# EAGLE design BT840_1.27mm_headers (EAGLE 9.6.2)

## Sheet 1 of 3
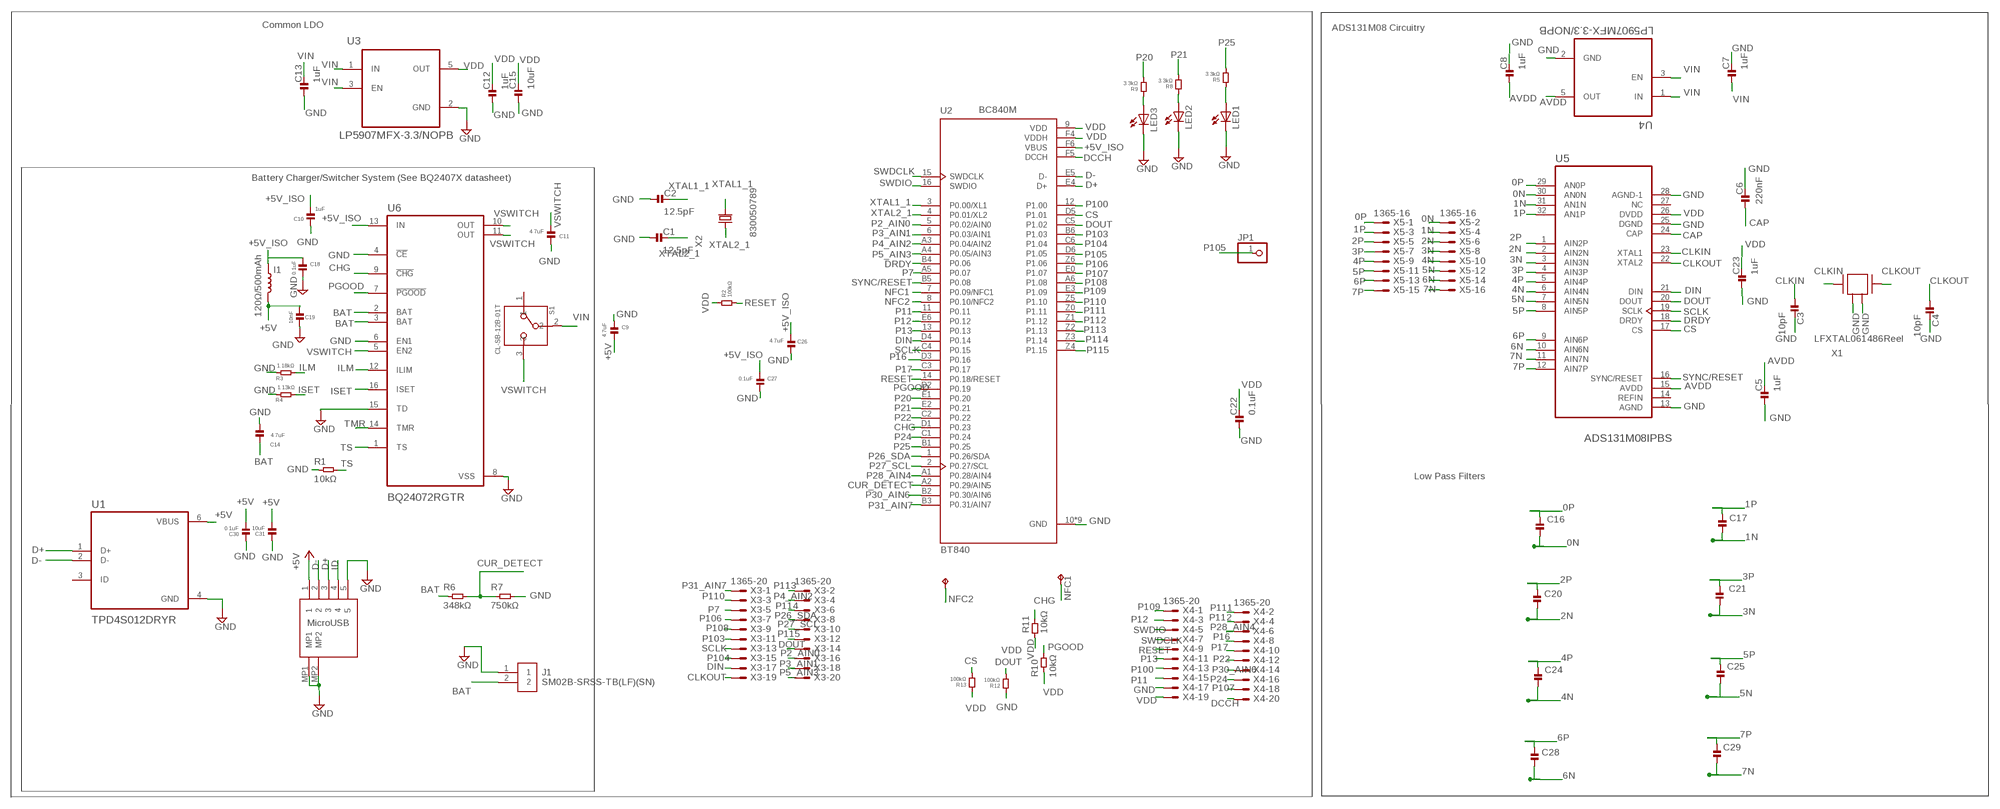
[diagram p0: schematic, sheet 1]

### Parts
C1  12.5pF  CAPACITOR.0201  [0201]
C2  12.5pF  CAPACITOR.0201  [0201]
C3  10pF  CAPACITOR.0201  [0201]
C4  10pF  CAPACITOR.0201  [0201]
C5  1uF  CAPACITOR.0201  [0201]
C6  220nF  CAPACITOR.0201  [0201]
C7  1uF  CAPACITOR.0201  [0201]
C8  1uF  CAPACITOR.0201  [0201]
C9  4.7uF  CAPACITOR.0201  [0201]
C10  1uF  CAPACITOR.0201  [0201]
C11  4.7uF  CAPACITOR.0201  [0201]
C12  1uF  CAPACITOR.0201  [0201]
C13  1uF  CAPACITOR.0201  [0201]
C14  4.7uF  CAPACITOR.0201  [0201]
C15  10uF  CAPACITOR.0402  [0402]
C16  100pF  CAPACITOR.0201  [0201]
C17  100pF  CAPACITOR.0201  [0201]
C18  0.1uF  CAPACITOR.0201  [0201]
C19  10nF  CAPACITOR.0201  [0201]
C20  100pF  CAPACITOR.0201  [0201]
C21  100pF  CAPACITOR.0201  [0201]
C22  0.1uF  CAPACITOR.0201  [0201]
C23  1uF  CAPACITOR.0201  [0201]
C24  100pF  CAPACITOR.0201  [0201]
C25  100pF  CAPACITOR.0201  [0201]
C26  4.7uF  CAPACITOR.0201  [0201]
C27  0.1uF  CAPACITOR.0201  [0201]
C28  100pF  CAPACITOR.0201  [0201]
C29  100pF  CAPACITOR.0201  [0201]
C30  0.1uF  CAPACITOR.0201  [0201]
C31  10uF  CAPACITOR.0402  [0402]
I1  120Ω/500mAh  12NH-0402  [0402_COILCRAFT]
J1  SM02B-SRSS-TB(LF)(SN)  [SM02B-SRSS-TB(LF)(SN)]
JP1  PINHD-1X1  [1X01]
LED1  LEDCHIPLED_0603  [CHIPLED_0603]
LED2  LEDCHIPLED_0603  [CHIPLED_0603]
LED3  LEDCHIPLED_0603  [CHIPLED_0603]
NFC1  TPTP14SQ  [TP14SQ]
NFC2  TPTP14SQ  [TP14SQ]
R1  10kΩ  RESISTOR.0201  [0201]
R2  100kΩ  RESISTOR.0201  [0201]
R3  1.18kΩ  RESISTOR.0201  [0201]
R4  1.13kΩ  RESISTOR.0201  [0201]
R5  3.3kΩ  RESISTOR.0201  [0201]
R6  348kΩ  RESISTOR.0201  [0201]
R7  750kΩ  RESISTOR.0201  [0201]
R8  3.3kΩ  RESISTOR.0201  [0201]
R9  3.3kΩ  RESISTOR.0201  [0201]
R10  10kΩ  RESISTOR.0402  [0402]
R11  10kΩ  RESISTOR.0402  [0402]
R12  100kΩ  RESISTOR.0402  [0402]
R13  100kΩ  RESISTOR.0402  [0402]
S1  CL-SB-12B-01T  [CL-SB-12B]
U1  TPD4S012DRYR  [PSON50P145X100X60-6N]
U2  BT840  [XCVR_BT840]
U3  LP5907MFX-3.3/NOPB  [SOT95P280X145-5N]
U4  LP5907MFX-3.3/NOPB  [SOT95P280X145-5N]
U5  ADS131M08IPBS  [QFP50P700X700X120-32N]
U6  BQ24072RGTR  [QFN50P300X300X100-17N]
U7  DX4R005JJ2R1800  [DX4R005JJ2R1800]
X1  ABM3B-8.000MHZ-B2-T  [ABM3B-8.000MHZ-B2-T]
X2  FC-12M  [FC-12M]
X3  1365-20  [1365-20]
X4  1365-20  [1365-20]
X5  1365-16  [1365-16]

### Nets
0N: C16.2 U5.30(AN0N) X5.2
0P: C16.1 U5.29(AN0P) X5.1
1N: C17.2 U5.31(AN1N) X5.4
1P: C17.1 U5.32(AN1P) X5.3
2N: C20.2 U5.2(AIN2N) X5.6
2P: C20.1 U5.1(AIN2P) X5.5
3N: C21.2 U5.3(AIN3N) X5.8
3P: C21.1 U5.4(AIN3P) X5.7
4N: C24.2 U5.6(AIN4N) X5.10
4P: C24.1 U5.5(AIN4P) X5.9
5N: C25.2 U5.7(AIN5N) X5.12
5P: C25.1 U5.8(AIN5P) X5.11
6N: C28.2 U5.10(AIN6N) X5.14
6P: C28.1 U5.9(AIN6P) X5.13
7N: C29.2 U5.11(AIN7N) X5.16
7P: C29.1 U5.12(AIN7P) X5.15
+5V: C9.2 C19.2 C30.2 C31.2 I1.P$2 U1.6(VBUS) U7.1
+5V_ISO: C10.2 C18.1 C26.2 C27.2 I1.P$1 U2.F6(VBUS) U6.13(IN)
AVDD: C5.2 C8.1 U4.5(OUT) U5.15(AVDD)
BAT: C14.2 J1.2 R6.1 U6.2(BAT) U6.3(BAT)
CAP: C6.1 U5.24(CAP)
CHG: R11.2 U2.D1(P0.23) U6.9(!CHG)
CLKIN: C3.1 U5.23(XTAL1) X1.1
CLKOUT: C4.1 U5.22(XTAL2) X1.3 X3.19
CS: R13.1 U2.D5(P1.01) U5.17(CS)
CUR_DETECT: R6.2 R7.1 U2.A2(P0.29/AIN5)
D+: U1.1(D+) U2.E4(D+) U7.3
D-: U1.2(D-) U2.E5(D-) U7.2
DCCH: U2.F5(DCCH) X4.20
DIN: U2.D4(P0.14) U5.21(DIN) X3.17
DOUT: R12.1 U2.C5(P1.02) U5.20(DOUT) X3.14
DRDY: U2.B4(P0.06) U5.18(DRDY)
GND: C1.1 C2.1 C3.2 C4.2 C5.1 C6.2 C7.2 C8.2 C9.1 C10.1 C11.1 C12.1 C13.1 C14.1 C15.1 C18.2 C19.1 C22.1 C23.1 C26.1 C27.1 C30.1 C31.1 J1.1 LED1.C LED2.C LED3.C R1.1 R3.1 R4.1 R7.2 R12.2 U1.4(GND) U2.10(GND) U2.A0(GND) U2.B0(GND) U2.C0(GND) U2.D0(GND) U2.F0(GND) U2.F1(GND) U2.F2(GND) U2.F3(GND) U3.2(GND) U4.2(GND) U5.13(AGND) U5.25(DGND) U5.28(AGND-1) U6.4(!CE) U6.6(EN1) U6.8(VSS) U6.15(TD) U7.5 U7.MP1 U7.MP2 X1.2 X1.4 X4.17
ID: U7.4
ILM: R3.2 U6.12(ILIM)
ISET: R4.2 U6.16(ISET)
LED1: LED1.A R5.2
LED2: LED2.A R8.2
LED3: LED3.A R9.2
NFC1: NFC2.TP U2.7(P0.09/NFC1)
NFC2: NFC1.TP U2.8(P0.10/NFC2)
P2_AIN0: U2.5(P0.02/AIN0) X3.16
P3_AIN1: U2.6(P0.03/AIN1) X3.18
P4_AIN2: U2.A3(P0.04/AIN2) X3.4
P5_AIN3: U2.A4(P0.05/AIN3) X3.20
P7: U2.A5(P0.07) X3.5
P11: U2.11(P0.11) X4.15
P12: U2.E6(P0.12) X4.3
P13: U2.13(P0.13) X4.11
P16: U2.D3(P0.16) X4.8
P17: U2.C3(P0.17) X4.10
P20: R9.1 U2.E1(P0.20)
P21: R8.1 U2.E2(P0.21)
P22: U2.C2(P0.22) X4.12
P24: U2.C1(P0.24) X4.16
P25: R5.1 U2.B1(P0.25)
P26_SDA: U2.1(P0.26/SDA) X3.8
P27_SCL: U2.2(P0.27/SCL) X3.10
P28_AIN4: U2.A1(P0.28/AIN4) X4.6
P30_AIN6: U2.B2(P0.30/AIN6) X4.14
P31_AIN7: U2.B3(P0.31/AIN7) X3.1
P100: U2.12(P1.00) X4.13
P103: U2.B6(P1.03) X3.11
P104: U2.C6(P1.04) X3.15
P105: JP1.1 U2.D6(P1.05)
P106: U2.Z6(P1.06) X3.7
P107: U2.E0(P1.07) X4.18
P108: U2.A6(P1.08) X3.9
P109: U2.E3(P1.09) X4.1
P110: U2.Z5(P1.10) X3.3
P111: U2.Z0(P1.11) X4.2
P112: U2.Z1(P1.12) X4.4
P113: U2.Z2(P1.13) X3.2
P114: U2.Z3(P1.14) X3.6
P115: U2.Z4(P1.15) X3.12
PGOOD: R10.2 U2.D2(P0.19) U6.7(!PGOOD)
RESET: R2.1 U2.14(P0.18/RESET) X4.9
SCLK: U2.C4(P0.15) U5.19(SCLK) X3.13
SWDCLK: U2.15(SWDCLK) X4.7
SWDIO: U2.16(SWDIO) X4.5
SYNC/RESET: U2.B5(P0.08) U5.16(SYNC/RESET)
TMR: U6.14(TMR)
TS: R1.2 U6.1(TS)
VDD: C12.2 C15.2 C22.2 C23.2 R2.2 R10.1 R11.1 R13.2 U2.9(VDD) U2.F4(VDDH) U3.5(OUT) U5.26(DVDD) X4.19
VIN: C7.1 C13.2 S1.2 U3.1(IN) U3.3(EN) U4.1(IN) U4.3(EN)
VSWITCH: C11.2 S1.3 U6.5(EN2) U6.10(OUT) U6.11(OUT)
XTAL1_1: C2.2 U2.3(P0.00/XL1) X2.2
XTAL2_1: C1.2 U2.4(P0.01/XL2) X2.1
Unconnected: S1.1 U1.3(ID) U5.14(REFIN) U5.27(NC)

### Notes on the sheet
- Common LDO
- ADS131M08 Circuitry
- BC840M
- Battery Charger/Switcher System (See BQ2407X datasheet)
- 830050789
- LFXTAL061486Reel
- Low Pass Filters
- MicroUSB

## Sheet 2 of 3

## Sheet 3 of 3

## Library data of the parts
C1-C31 = standardparts:CAPACITOR
I1 = spkfncoils:12NH; MOUSER_PART: 994-0402HP-12NXGLU; PROD_ID: NDUC-15271; VALUE: 12nH
J1 = SM02B-SRSS-TB_LF__SN_:SM02B-SRSS-TB(LF)(SN): JST (JAPAN SOLDERLESS TERMINALS) - SM02B-SRSS-TB (LF)(SN) - HEADER, R/A, 2WAY; AVAILABILITY: In Stock; DESCRIPTION: Connector Header Surface Mount, Right Angle 2 position 0.039 (1.00mm); MF: JST Sales; MP: SM02B-SRSS-TB(LF)(SN); PACKAGE: None; PRICE: None
JP1 = pinhead:PINHD-1X1: PIN HEADER
LED1-LED3 = adafruit:LED: LED
NFC1 NFC2 = testpad:TP: Test pad
R1 R2 R4-R13 = standardparts:RESISTOR
R3 = standardparts:RESISTOR; SPICEPREFIX: R
S1 = CL-SB-12B-01T:CL-SB-12B-01T: Check prices; AVAILABILITY: In Stock; DESCRIPTION: Slide Switch SPDT Surface Mount; MF: Nidec Copal; MP: CL-SB-12B-01T; PACKAGE: None; PRICE: None
U1 = TPD4S012DRYR:TPD4S012DRYR: Check prices; AVAILABILITY: In Stock; DESCRIPTION: 4-channel USB ESD solution with power clamp 6-SON -40 to 85; MF: Texas Instruments; MP: TPD4S012DRYR; PACKAGE: USON-6 Texas Instruments; PRICE: None; PURCHASE-URL: https://pricing.snapeda.com/search/part/TPD4S012DRYR/?ref=eda
U2 = BT840:BT840: Bluetooth LE Module, Nordic nRF52840 SoC, Range 180 meters Check availability; AVAILABILITY: In Stock; DESCRIPTION: 802.15.4, Bluetooth Bluetooth v5.0, Thread, Zigbee® Transceiver Module 2.4GHz Antenna Not Included, U.FL Surface Mount; MF: Fanstel Corp.; MP: BT840; PACKAGE: SMD-16 Fanstel Corp.; PRICE: None; PURCHASE-URL: https://pricing.snapeda.com/search/part/BT840/?ref=eda
U3 U4 = LP5907MFX-3.3_NOPB:LP5907MFX-3.3/NOPB: IC REG LINEAR 3.3V 250MA SOT23; AVAILABILITY: Unavailable; DESCRIPTION: Linear Voltage Regulator IC 1 Output 250mA SOT-23-5; MF: Texas Instruments; MP: LP5907MFX-3.3/NOPB; PACKAGE: SOT-23 Texas Instruments; PRICE: None
U5 = ADS131M08IPBS:ADS131M08IPBS: None Check prices; AVAILABILITY: Warning; DESCRIPTION: 24-bit 32-kSPS 8-channelsimultaneous-sampling delta-sigma ADC 32-TQFP -40 to 125; MF: Texas Instruments; MP: ADS131M08IPBS; PACKAGE: TQFP-32 Texas Instruments; PRICE: None; PURCHASE-URL: https://pricing.snapeda.com/search/part/ADS131M08IPBS/?ref=eda
U6 = BQ24072RGTR:BQ24072RGTR: Check prices; AVAILABILITY: In Stock; DESCRIPTION: Standalone 1-cell 1.5-A linear charger, Power Path, 4.2-V VBAT and VOUT=VBAT + 225mV 16-VQFN -40 to 85; MF: Texas Instruments; MP: BQ24072RGTR; PACKAGE: VQFN-16 Texas Instruments; PRICE: None; PURCHASE-URL: https://pricing.snapeda.com/search/part/BQ24072RGTR/?ref=eda
U7 = DX4R005JJ2R1800:DX4R005JJ2R1800: Check prices; AVAILABILITY: In Stock; DESCRIPTION: USB - micro B USB 2.0 Receptacle Connector 5 Position Surface Mount, Right Angle; Through Hole; MF: JAE Electronics; MP: DX4R005JJ2R1800; PACKAGE: None; PRICE: None
X1 = Crystals_Oscillators:ABM3B-8.000MHZ-B2-T: CRYSTAL 8.0000MHZ 18PF SMD Manufacturer's datasheet; CREATED_BY: PCBLayout.com; DIGIKEY_PART_NUMBER: 535-9720-2-ND; MANUFACTURER: Abracon LLC; MPN: ABM3B-8.000MHZ-B2-T; PACKAGE: SMD 4
X2 = crystal:FC-12M: kHz RANGE CRYSTAL UNIT
X3 X4 = con-leotronics:1365-20: DUAL ROW STRAIGHT HEADER 1364 SERIES. 1.27mm x 1.27mm. Without Fixing Post. SMT Source: http://www.leotronics.co.uk/Conexcon/Data%20Sheets/sec.%20A/1364ing.pdf; OC_FARNELL: unknown; OC_NEWARK: unknown
X5 = con-leotronics:1365-16: DUAL ROW STRAIGHT HEADER 1364 SERIES. 1.27mm x 1.27mm. Without Fixing Post. SMT Source: http://www.leotronics.co.uk/Conexcon/Data%20Sheets/sec.%20A/1364ing.pdf; OC_FARNELL: unknown; OC_NEWARK: unknown

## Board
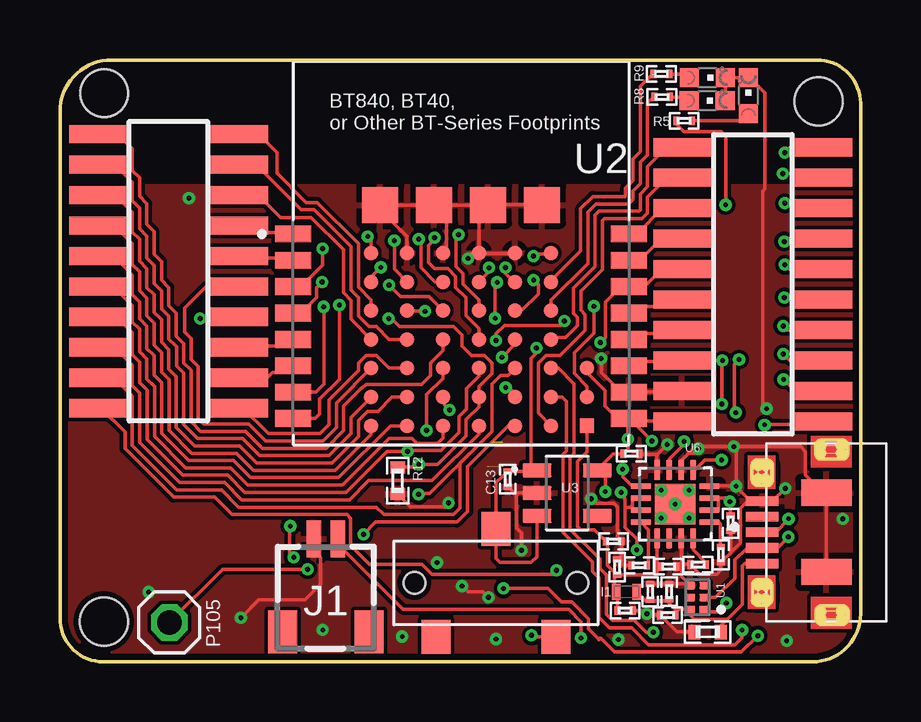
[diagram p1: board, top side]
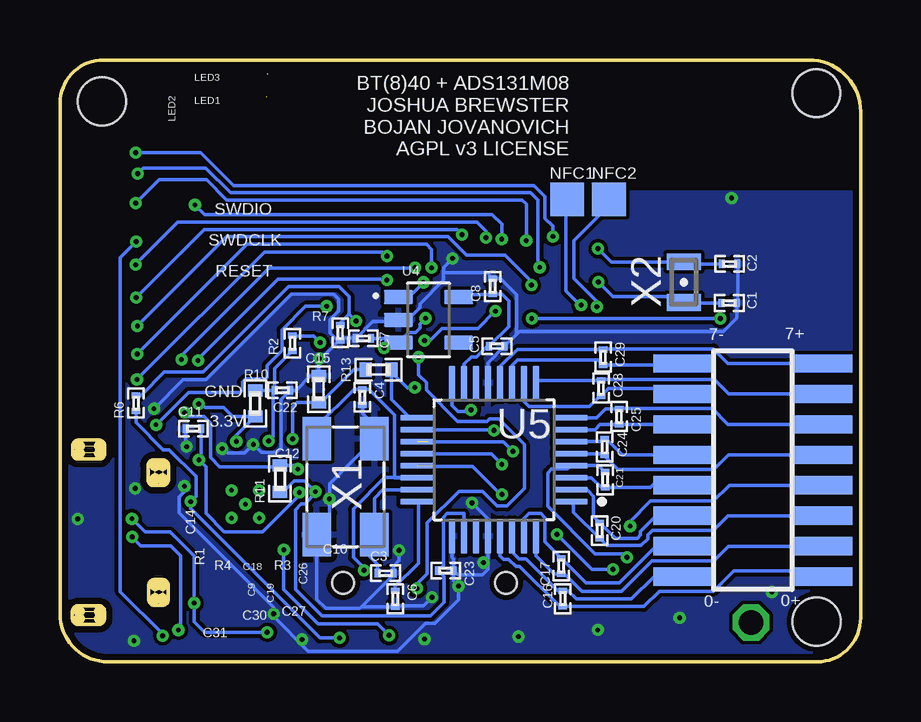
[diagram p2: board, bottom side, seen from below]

Size 33.38 x 25.1 mm. Coordinates in mm from the lower left corner, seen from the top.
Outline: 31.75,1.56 arc-90 31.52,1.79 31.52,2.1 arc-90 31.75,2.34 32.62,2.34 arc-90 32.85,2.1 32.85,1.79 arc-90 32.63,1.56 31.75,1.56
Outline: 31.74,8.45 arc-90 31.51,8.68 31.51,8.98 arc-90 31.74,9.25 32.62,9.25 arc-90 32.84,8.98 32.84,8.68 arc-90 32.62,8.45 31.74,8.45
Outline: 29.67,2.59 arc-90 29.44,2.36 29.1,2.36 arc-90 28.87,2.59 28.87,3.2 arc-90 29.1,3.43 29.44,3.43 arc-90 29.67,3.2 29.67,2.59
Outline: 29.7,7.58 arc-90 29.47,7.35 29.13,7.35 arc-90 28.85,7.58 28.85,8.2 arc-90 29.13,8.42 29.47,8.42 arc-90 29.7,8.19 29.7,7.58
Outline: 33.38,2.01 arc-90 31.37,0 1.8,0 arc-90 0,1.83 0,22.94 arc-90 2.16,25.1 31.55,25.1 arc-90 33.38,23.29 33.38,2.01
Copper layers (1*16): Top 0.035mm / dielectric 1.5mm / Bottom 0.035mm
Design rules "default *": minimum track width 4mil, minimum drill 0.2mm, track to track 6mil, track to pad 6mil, pad to pad 6mil, via to via 6mil, smd to smd 6mil, copper to edge 10mil, drill to drill 6mil, minimum pad ring 6mil, minimum via ring 6mil, stop-mask expansion 4mil, vias tented up to drill 20mil, thermal gap 10mil
Holes 2 mm at 1.84,23.71 31.62,23.36 1.83,1.67

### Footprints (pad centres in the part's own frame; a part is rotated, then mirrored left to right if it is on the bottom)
0201 = smd 0.25 x 0.35: 1 -0.325,0; 2 0.325,0
0402 = smd 0.5 x 0.6: 1 -0.55,0; 2 0.55,0
0402_COILCRAFT = smd 0.356 x 0.66: P$1 -0.432,0; P$2 0.432,0
SM02B-SRSS-TB(LF)(SN) = smd 0.6 x 1.55: 1 -0.5,1.975; 2 0.5,1.975 | smd 1.2 x 1.8: 3 -1.8,-1.9; 4 1.8,-1.9
1X01 = drill 1.016 octagon: 1 0,0
CHIPLED_0603 = smd 0.8 x 0.8: A 0,-0.75; C 0,0.75
TP14SQ = smd 1.4 x 1.4: TP 0,0
CL-SB-12B = smd 1.2 x 1.4: 1 -2.5,-2.25; 2 0,2.25; 3 2.5,-2.25 | hole 0.9: 3.4,0; -3.4,0
PSON50P145X100X60-6N = smd 0.42 x 0.3: 1 -0.29,0.5 | smd 0.41 x 0.3: 2 -0.295,0; 3 -0.295,-0.5; 4 0.295,-0.5; 5 0.295,0; 6 0.295,0.5
XCVR_BT840 = smd 1.5 x 0.7: 1 -7,0.8; 2 -7,-0.3; 3 -7,-1.4; 4 -7,-2.5; 5 -7,-3.6; 6 -7,-4.7; 7 -7,-5.8; 8 -7,-6.9; 9 7,-6.9; 10 7,-5.8; 11 7,-4.7; 12 7,-3.6; 13 7,-2.5; 14 7,-1.4; 15 7,-0.3; 16 7,0.8 | smd 0.6 x 0.6: A0 -2.25,0; A1 -2.25,-1.2; A2 -2.25,-2.4; A3 -2.25,-3.6; A4 -2.25,-4.8; A5 -2.25,-6; A6 -2.25,-7.2; B0 -0.75,0; B1 -0.75,-1.2; B2 -0.75,-2.4; B3 -0.75,-3.6; B4 -0.75,-4.8; B5 -0.75,-6; B6 -0.75,-7.2; C0 0.75,0; C1 0.75,-1.2; C2 0.75,-2.4; C3 0.75,-3.6; C4 0.75,-4.8; C5 0.75,-6; C6 0.75,-7.2; D0 2.25,0; D1 2.25,-1.2; D2 2.25,-2.4; D3 2.25,-3.6; D4 2.25,-4.8; D5 2.25,-6; D6 2.25,-7.2; E0 3.75,0; E1 3.75,-1.2; E2 3.75,-2.4; E3 3.75,-3.6; E4 3.75,-4.8; E5 3.75,-6; E6 3.75,-7.2; F4 5.25,-4.8; F5 5.25,-6; F6 5.25,-7.2; Z0 -3.75,0; Z1 -3.75,-1.2; Z2 -3.75,-2.4; Z3 -3.75,-3.6; Z4 -3.75,-4.8; Z5 -3.75,-6; Z6 -3.75,-7.2 | smd 1.5 x 1.5: F0 -3.375,2; F1 -1.125,2; F2 1.125,2; F3 3.375,2
SOT95P280X145-5N = smd 1.21 x 0.59: 1 -1.255,0.95; 2 -1.255,0; 3 -1.255,-0.95; 4 1.255,-0.95; 5 1.255,0.95
QFP50P700X700X120-32N = smd 1.44 x 0.26: 1 -3.195,1.75; 2 -3.195,1.25; 3 -3.195,0.75; 4 -3.195,0.25; 5 -3.195,-0.25; 6 -3.195,-0.75; 7 -3.195,-1.25; 8 -3.195,-1.75; 17 3.195,-1.75; 18 3.195,-1.25; 19 3.195,-0.75; 20 3.195,-0.25; 21 3.195,0.25; 22 3.195,0.75; 23 3.195,1.25; 24 3.195,1.75 | smd 0.26 x 1.44: 9 -1.75,-3.195; 10 -1.25,-3.195; 11 -0.75,-3.195; 12 -0.25,-3.195; 13 0.25,-3.195; 14 0.75,-3.195; 15 1.25,-3.195; 16 1.75,-3.195; 25 1.75,3.195; 26 1.25,3.195; 27 0.75,3.195; 28 0.25,3.195; 29 -0.25,3.195; 30 -0.75,3.195; 31 -1.25,3.195; 32 -1.75,3.195
QFN50P300X300X100-17N = smd 0.86 x 0.26: 1 -1.435,0.75; 2 -1.435,0.25; 3 -1.435,-0.25; 4 -1.435,-0.75; 9 1.435,-0.75; 10 1.435,-0.25; 11 1.435,0.25; 12 1.435,0.75 | smd 0.26 x 0.86: 5 -0.75,-1.435; 6 -0.25,-1.435; 7 0.25,-1.435; 8 0.75,-1.435; 13 0.75,1.435; 14 0.25,1.435; 15 -0.25,1.435; 16 -0.75,1.435 | smd 1.68 x 1.68: 17 0,0 | drill 0.2 pad 0.4: 18 0,0; 19 -0.58,0.58; 20 0.58,0.58; 21 -0.58,-0.58; 22 0.58,-0.58
DX4R005JJ2R1800 = smd 1.35 x 0.4: 1 1.525,1.3; 2 1.525,0.65; 3 1.525,0; 4 1.525,-0.65; 5 1.525,-1.3 | smd 2.1 x 1.1: MP1 -1.15,1.65; MP2 -1.15,-1.65
ABM3B-8.000MHZ-B2-T = smd 1.8 x 1.2: 1 -2,-1.2; 2 2,-1.2; 3 2,1.2; 4 -2,1.2
FC-12M = smd 0.7 x 1.4: 1 -0.85,0; 2 0.85,0
1365-20 = smd 0.76 x 2.4: 1 -5.715,-2.95; 2 -5.715,2.95; 3 -4.445,-2.95; 4 -4.445,2.95; 5 -3.175,-2.95; 6 -3.175,2.95; 7 -1.905,-2.95; 8 -1.905,2.95; 9 -0.635,-2.95; 10 -0.635,2.95; 11 0.635,-2.95; 12 0.635,2.95; 13 1.905,-2.95; 14 1.905,2.95; 15 3.175,-2.95; 16 3.175,2.95; 17 4.445,-2.95; 18 4.445,2.95; 19 5.715,-2.95; 20 5.715,2.95
1365-16 = smd 0.76 x 2.4: 1 -4.445,-2.95; 2 -4.445,2.95; 3 -3.175,-2.95; 4 -3.175,2.95; 5 -1.905,-2.95; 6 -1.905,2.95; 7 -0.635,-2.95; 8 -0.635,2.95; 9 0.635,-2.95; 10 0.635,2.95; 11 1.905,-2.95; 12 1.905,2.95; 13 3.175,-2.95; 14 3.175,2.95; 15 4.445,-2.95; 16 4.445,2.95

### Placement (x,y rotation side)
C1  5.47,14.96 180 bottom
C2  5.46,16.59 180 bottom
C3  19.8,3.69 0 bottom
C4  20.77,11.04 270 bottom
C5  15.16,13.16 180 bottom
C6  19.4,2.63 270 bottom
C7  20.73,13.48 180 bottom
C8  15.33,15.65 90 bottom
C9  25.4,2.92 270 top
C10  23.09,5.02 180 top
C11  27.81,9.72 0 bottom
C12  23.82,8.68 180 top
C13  18.67,7.61 90 top
C14  27.95,5.78 90 top
C15  22.59,11.37 270 bottom
C16  12.41,2.63 90 bottom
C17  12.48,4 90 bottom
C18  25.37,3.97 0 top
C19  24.61,2.92 270 top
C20  10.87,5.47 90 bottom
C21  10.65,7.59 270 bottom
C22  24.1,11.32 180 bottom
C23  17.29,3.8 180 bottom
C24  10.66,8.96 90 bottom
C25  10.07,10.23 270 bottom
C26  23.23,3.95 270 top
C27  23.56,2.14 180 top
C28  10.82,11.41 270 bottom
C29  10.74,12.7 270 bottom
C30  25.34,1.95 0 top
C31  27.01,1.24 0 top
I1  23.61,2.92 0 top
J1  11.08,3.15 0 top
JP1  4.56,1.64 0 top
LED1  28.7,23.61 0 top
LED2  26.98,23.4 270 top
LED3  26.99,24.36 270 top
NFC1  12.22,19.28 0 bottom
NFC2  10.49,19.28 0 bottom
R1  27.55,4.46 90 top
R2  23.68,13.28 270 bottom
R3  24.15,4.02 0 top
R4  26.6,4.06 0 top
R5  26.02,22.56 0 top
R6  30.2,10.79 90 bottom
R7  21.69,13.72 270 bottom
R8  25.1,23.55 0 top
R9  25.07,24.51 0 top
R10  25.24,10.77 270 bottom
R11  24.2,7.63 90 bottom
R12  14.08,7.55 270 top
R13  20.1,12.18 180 bottom
S1  18.17,3.29 0 top
U1  26.57,2.68 180 top
U2  16.72,17.04 0 top
U3  21.15,7.04 0 top
U4  18.01,14.26 0 bottom
U5  15.28,8.43 180 bottom
U6  25.65,6.57 180 top
U7  30.8,5.4 180 top
X1  21.47,7.3 90 bottom
X2  7.37,15.83 90 bottom
X3  4.53,16.29 270 top
X4  28.89,15.74 270 top
X5  4.49,8 90 bottom

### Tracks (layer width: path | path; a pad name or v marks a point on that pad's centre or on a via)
0N
  Bottom 0.152: X5.2 8.62,3.55 9.55,2.62 11.85,2.62 12.19,2.95 C16.2 12.61,2.95 13.94,4.28 14.24,4.28 14.54,4.58 U5.30
0P
  Bottom 0.152: X5.1 1.78,3.8 5.29,3.8 6.14,2.94 8.4,2.94 9.03,2.3 C16.1 | C16.1 12.45,2.34 | C16.1 12.54,2.3 14.21,3.97 14.36,3.97 14.67,4.28 14.89,4.28 15.03,4.42 U5.29
1N
  Bottom 0.152: X5.4 8.53,4.82 10.05,3.3 11.45,3.3 C17.2 13.15,5 13.15,6.01 13.33,6.18 13.82,6.18 14.03,5.97 U5.31
1P
  Bottom 0.152: U5.32 13.53,4.42 12.78,3.67 C17.1 12.35,3.67 11.61,2.93 9.97,2.93 8.69,4.21 6.12,4.21 5.51,4.82 X5.3
2N
  Bottom 0.152: U5.2 12.05,7.14 11.37,7.14 11.14,6.91 11.14,6.07 C20.2 10.23,5.15 9.31,5.15 9.17,5.3 9.17,5.45 8.52,6.09 X5.6
2P
  Bottom 0.152: X5.5 5.53,6.09 6.14,5.48 8.68,5.48 8.86,5.3 8.86,5.13 9.15,4.85 10.57,4.85 C20.1 11.96,6.24 11.96,6.55 U5.1
3N
  Bottom 0.152: X5.8 7.62,7.54 8.49,7.54 8.77,7.26 C21.2 | 10.61,7.26 C21.2 | U5.3 11.21,7.68 10.79,7.26 C21.2
3P  (via drill 0.2)
  Top 0.152: v9.75,4.36 9.57,4.53 9.57,5.62 v9.6,5.66
  Bottom 0.152: X5.7 5.47,7.36 6.13,6.7 8.77,6.7 9.6,5.86 v9.6,5.66 | C21.1 10.92,8.18 U5.4 12.23,8.04 12.88,8.04 13.04,7.88 13.04,6.47 11.07,4.51 9.9,4.51 v9.75,4.36
4N
  Bottom 0.152: U5.6 10.83,9.19 10.73,9.28 C24.2 10.58,9.28 9.93,8.63 X5.10
4P
  Bottom 0.152: X5.9 5.52,8.63 6.12,8.02 10.11,8.02 10.69,8.61 C24.1 10.71,8.68 U5.5
5N
  Bottom 0.152: U5.7 11.08,9.68 10.86,9.9 C25.2 X5.12
5P
  Bottom 0.152: X5.11 5.52,9.9 6.18,10.56 10.05,10.56 C25.1 10.63,10.55 11,10.18 U5.8
6N
  Bottom 0.152: X5.14 7.66,11.39 10.51,11.39 C28.2 10.87,11.09 11.31,10.65 13.83,10.65 14.03,10.86 U5.10
6P
  Bottom 0.152: X5.13 5.5,11.17 6.1,11.78 10.78,11.78 C28.1 13.42,11.74 U5.9
7N
  Bottom 0.152: U5.11 14.53,12.36 14.3,12.59 10.95,12.59 C29.2 7.5,12.38 X5.16
7P
  Bottom 0.152: U5.12 15.03,12.31 14.31,13.03 C29.1 10.72,13.05 6.13,13.05 5.52,12.44 X5.15
+5V
  Top 0.152: U7.1 28.54,4.1 28.44,4 28.44,2.4 27.82,1.78 | 27.82,1.78 26.44,1.78 26.27,1.95 U1.6 25.66,2.18 | 25.66,2.18 25.75,2.1 25.66,2.02 C30.2 | 25.66,2.18 25.4,2.45 | 25.4,2.45 25.3,2.55 24.66,2.55 | 24.66,2.55 24.41,2.55 I1.P$2 | 25.4,2.45 C9.2 | C19.2 24.66,2.55 | C31.2 27.56,1.51 27.82,1.78
+5V_ISO
  Top 0.152: U6.13 24.89,4.06 | 24.89,4.06 24.89,3.62 C26.2 | U2.F6 21.97,8.75 21.57,8.35 21.57,5.66 21.72,5.51 22.27,5.51 C10.2 22.82,4.96 22.82,4.01 23.21,3.62 C26.2 | C18.1 24.95,4.06 24.89,4.06 | C26.2 23.12,3.51 23.12,2.98 I1.P$1 23.24,2.86 C27.2
AVDD
  Bottom 0.152: U4.5 16.64,15.32 C8.1 14.96,15.33 14.66,15.04 14.66,13.98 C5.2 15.56,13.16 16.01,12.72 16.22,12.72 16.53,12.41 U5.15
BAT  (via drill 0.2)
  Top 0.152: U6.2 27.45,6.32 27.45,6.81 27.43,6.82 | J1.2 11.63,5.12 11.65,5.1 11.65,4.84 14.3,2.19 21.21,2.19 21.72,1.68 v21.72,0.99 | 27.43,6.82 U6.3 | C14.2 27.95,6.65 v27.93,6.68 27.77,6.84 27.41,6.84 27.43,6.82
  Bottom 0.152: v21.72,0.99 22.53,0.99 27.93,6.39 v27.93,6.68 27.71,6.9 27.71,7.73 28.82,8.84 29.06,8.84 30.2,9.98 R6.1
CAP
  Bottom 0.152: U5.24 18.43,6.63 18.43,4.11 19.4,3.14 C6.1
CHG  (via drill 0.2)
  Top 0.152: U6.9 23.85,7.32 23.46,7.71 v23.46,8.03 v23.46,8.04 | 19.07,15.87 18.94,15.87 | v18.58,16.43 18.58,16.19 18.86,15.91 18.9,15.91 18.94,15.87 | v28.31,12.61 28.12,12.41 28.12,10.44 v28.17,10.39 v28.18,10.39 | U2.D1 18.94,15.87
  Bottom 0.152: v23.46,8.04 23.61,8.18 R11.2 24.25,8.13 26.71,8.13 27.1,8.52 27.1,9.96 27.37,10.24 28.02,10.24 v28.18,10.39 | v18.58,16.43 18.59,16.42 24.66,16.42 28.39,12.69 v28.31,12.61
CLKIN
  Bottom 0.152: U5.23 19.92,7.17 20.27,6.82 X1.1 20.46,5.11 20.46,4.4 20.13,4.07 C3.1
CLKOUT  (via drill 0.2)
  Top 0.152: v20.7,3.81 20.55,3.66 15.51,3.66 15.1,4.07 12.9,4.07 12.12,4.85 12.12,5.99 11.97,6.14 7.18,6.14 6.45,6.87 4.73,6.87 2.71,8.89 2.71,9.58 1.72,10.57 X3.19 2.12,10.57
  Bottom 0.152: X1.3 22.67,9.82 21.12,11.36 C4.1 20.48,11.36 19.43,10.3 19.43,7.68 U5.22 19.84,7.68 21.15,6.37 21.15,4.35 20.7,3.91 v20.7,3.81
CS  (via drill 0.2)
  Top 0.152: U2.D5 18.97,11.19 18.65,11.51 v18.58,11.44
  Bottom 0.152: U5.17 18.78,10.18 19.55,10.94 R13.1 19.55,12.07 18.89,11.41 18.61,11.41 v18.58,11.44
CUR_DETECT  (via drill 0.2)
  Top 0.152: v21.03,14.21 20.86,14.03 18.53,14.03 18.18,13.68 v18.18,13.4 | 15.01,14.61 v15.21,14.61 v15.21,14.62 14.49,14.62 U2.A2 14.45,14.64
  Bottom 0.152: R7.1 21.69,14.13 21.32,14.51 | R6.2 30,11.11 29.03,12.08 27.4,12.08 23.84,15.64 21.73,15.64 21.32,15.23 21.32,14.51 | 21.32,14.51 21.06,14.25 21.07,14.25 v21.03,14.21 | v18.18,13.4 17.96,13.4 17.45,13.91 15.95,13.91 15.24,14.62 v15.21,14.62
D+  (via drill 0.2)
  Top 0.152: U7.3 29.85,5.4 30.37,5.93 v30.37,5.97 | v27.78,2.45 27.42,2.09 26.95,2.09 U1.1 | U2.E4 20.78,12.24 21.43,11.59 21.43,8.66 21.26,8.5 21.26,5.53 22.51,4.28 22.51,3.89 22.77,3.63 22.77,1.98 23.02,1.73 23.96,1.73 24.44,1.24 v24.73,1.24 v24.73,1.23
  Bottom 0.152: v30.37,5.97 29.82,5.41 28.77,5.41 27.78,4.42 v27.78,2.45 27.78,1.67 27.34,1.23 v24.73,1.23
D-  (via drill 0.2)
  Top 0.152: U1.2 27.33,2.68 28.13,3.49 28.13,4.25 28.63,4.74 28.69,4.74 28.7,4.75 U7.2 29.92,4.75 v30.37,5.2 30.02,4.86 29.25,4.86 | U2.E5 20.92,11.04 21.11,10.85 21.11,8.8 20.96,8.64 20.96,5.55 20.96,5.41 22.21,4.16 22.21,3.76 22.47,3.5 22.47,1.85 22.91,1.41 23.84,1.41 24.54,0.71 28.14,0.71 28.44,1.01 v28.44,1.33
  Bottom 0.152: v28.44,1.33 28.35,1.41 28.35,4.42 28.77,4.84 30.01,4.84 v30.37,5.2
DCCH  (via drill 0.2)
  Top 0.152: U2.F5 21.97,11.49 21.44,12.02 21.44,12.9 22.25,13.71 v22.25,14.83 v22.26,14.83 | v29.37,9.88 v29.38,9.89 31.7,9.89 X4.20
  Bottom 0.152: v29.37,9.88 29.36,9.88 28.01,11.24 25.87,11.24 25.77,11.34 25.77,11.67 25.63,11.8 24.79,11.8 24.73,11.87 24.73,12.36 24.12,12.97 24.12,13.84 23.13,14.83 v22.26,14.83
DIN  (via drill 0.2)  (1 unrouted)
  Top 0.152: U2.D4 18.67,11.94 18.36,11.94 18,11.59 18,9.6 17.51,9.11 | 17.51,9.11 16.68,8.28 16.68,6.42 16.41,6.14 13.51,6.14 13.2,6.45 7.46,6.45 6.73,7.17 4.86,7.17 3.02,9.02 3.02,9.25 3.01,9.26 3.01,11.08 2.25,11.84 X3.17 | 17.51,9.11 15.41,7.01 14.98,7.01 v14.95,6.98
  Bottom 0.152: v14.95,6.98 15,6.98 16.18,8.16 17.82,8.16
DOUT  (via drill 0.2)
  Top 0.152: v13.7,14.31 13.81,14.31 14.15,13.98 16.41,13.98 16.76,13.63 16.76,13.18 17.16,12.77 17.69,12.77 18.01,12.45 18.01,12.03 17.47,11.49 U2.C5 17.47,10.63 16.94,10.1 16.94,9.41 15.74,8.22 14.97,8.22 v14.96,8.23 14.85,8.12 14.1,8.12 R12.1 | v5.85,14.32 5.86,14.3 6.37,14.3 6.45,14.38 X3.14
  Bottom 0.152: v14.96,8.23 15.39,8.67 U5.20 | v13.7,14.31 | v13.7,14.31 5.88,14.31 5.87,14.32 v5.85,14.32
DRDY  (via drill 0.2)
  Top 0.152: v15.28,9.65 15.29,9.66 15.29,11.14 15.97,11.82 U2.B4
  Bottom 0.152: U5.18 15.3,9.67 v15.28,9.65
GND  (via drill 0.2)
  Top 0.152: U6.15 25.9,4.06 | 25.9,4.06 25.9,3.56 U1.4 26.21,3.25 C9.1 C19.1 | U6.4 v28.19,7.32 | U7.5 28.78,6.7 28.19,7.29 v28.19,7.32 | v28.19,7.32 28.19,8.82 28.04,8.97 | 28.02,8.99 28.04,8.97 | U7.MP1 U7.MP2 31.83,7.05 31.08,7.8 31.08,8.01 31.07,8.01 31.07,8.77 30.87,8.97 28.04,8.97 | v22.56,12.65 22.57,12.63 22.57,12.07 23.39,11.24 U2.10 24.86,11.25 24.91,11.29 X4.17 | 19.44,7.04 U3.2 18.92,7.04 C13.1 | U6.8 24.89,8.64 v25.32,9.06 24.9,8.65 24.18,8.65 C12.1 | v22.15,6.79 22.33,6.61 23.09,6.61 23.24,6.46 23.24,5.12 23.34,5.02 C10.1 23.41,4.09 C26.1 23.48,4.02 R3.1 | 25.9,4.06 R4.1 26.67,3.65 27.38,3.65 27.55,3.83 27.55,4.07 | 25.9,4.06 25.78,4.06 C18.2 | 27.55,4.07 27.65,4.16 27.65,4.24 27.96,4.55 27.96,4.56 | 27.96,4.56 28.36,4.96 28.36,6.39 28.66,6.69 U7.5 | C27.1 24.33,2.14 v24.47,2 24.49,2 24.54,1.95 C30.1 25.72,1.24 C31.1 | 27.96,4.56 27.96,5.44 C14.1 | R1.1 27.55,4.07 | U6.6 25.91,8.02 25.91,8.4 26.22,8.71 26.44,8.71 v26.62,8.89 26.62,8.98 26.62,8.99 28.02,8.99 | 28.02,8.99 28.07,8.99 v28.09,8.97 | U2.A0 14.48,17.74 13.34,18.87 U2.F0 15.51,19.04 15.54,19.01 15.55,19 U2.F1 | U2.B0 16.11,17.19 16.11,18.52 U2.F1 | U2.F1 U2.F2 | 17.47,17.08 U2.C0 17.47,18.67 U2.F2 | U2.F3 20.08,19.06 U2.F2 | U2.F2 17.25,19.06 | U2.F2 | U2.D0 18.94,17.01 17.12,17.01 17.01,16.91 v17.01,16.82 | C13.1 | C13.1 19.02,6.93 19.02,5.59 19.24,5.38 v19.24,4.65 | v17.87,2.69 17.64,2.92 17,2.92 v16.76,3.16 | R12.2 14.61,6.47 16.05,6.47 v16.2,6.62 v16.2,6.63 | U7.5 29.7,6.7 v30.23,7.23 | J1.1 10.58,4.61 10.87,4.32 10.87,3.23 10.21,2.58 8.28,2.58 v7.54,1.83 | LED2.C 27.74,23.42 LED3.C LED1.C 28.77,24.36 29.39,23.74 29.39,19.71 29.3,19.62 29.3,10.7 v29.46,10.55
  Bottom 0.152: C4.2 20.77,10.36 20.21,9.8 20.21,9.36 X1.2 | C5.1 15.53,12.46 U5.13 | 17.39,16.22 15.57,16.22 C8.2 15.02,15.98 14.35,15.3 14.35,13.65 C5.1 | v28.19,7.32 28.19,7.1 28.41,6.88 28.41,6.2 24.47,2.27 v24.47,2 24.47,1.9 23.02,0.45 19.3,0.45 18.14,1.6 17.75,1.6 16.76,2.59 v16.76,3.16 16.97,3.37 C23.1 | 20.8,2.3 20.88,2.22 22.28,2.22 22.67,2.61 X1.4 22.15,5.82 v22.15,6.79 22.15,7.42 X1.2 | 20.8,2.3 19.48,3.62 C3.2 19.48,3.98 19.24,4.22 v19.24,4.65 | C5.1 14.83,13.15 | v25.32,9.06 25.32,9.03 | C11.1 28.14,9.02 v28.09,8.97 | v25.32,9.06 25.67,8.71 26.39,8.71 26.57,8.89 v26.62,8.89 | C2.1 5.11,16.57 5.11,15 C1.1 5.15,14.33 5.71,13.77 14.23,13.77 C5.1 | U5.25 17.04,5.22 17.04,4.36 16.97,4.29 C23.1 | v25.32,9.06 24.97,8.72 24.37,8.72 24.16,8.93 24.16,10.93 C22.1 23.54,11.32 22.94,11.92 C15.1 22.6,11.93 22.6,12.57 22.55,12.63 v22.56,12.65 22.49,12.65 21.74,13.39 R7.2 | R7.2 21.59,13.5 21.06,13.5 C7.2 20.34,14.18 19.34,14.18 U4.2 18.89,14.26 18.37,14.78 18.37,14.93 17.39,15.92 17.39,16.22 | X1.2 20.34,9.3 | 15.54,4.23 15.54,5.05 15.53,5.05 U5.28 15.53,5.97 v16.2,6.63 | 15.54,4.23 15.54,3.86 15.77,3.63 16.79,3.63 C23.1 | 20.8,2.3 C6.2 19.36,2.34 18.22,2.34 v17.87,2.69 | v17.01,16.82 17.39,16.45 17.39,16.22 | R7.2 21.81,13.39 22.12,13.71 22.12,14.27 21.77,14.62 21.77,15.13 21.97,15.33 23.71,15.33 27.28,11.77 28.23,11.77 v29.46,10.55 | 15.54,4.23 15.63,4.23 v15.72,4.14
  other vias: 3.7,2.91 5.38,19.34 14.27,1.05 30.29,0.87 32.63,5.95 23.28,0.93 18.18,0.95 10.96,1.33
  pour Top: 0.55,-0.98 -0.72,0.29 -0.72,19.34 -0.21,19.85 34.33,19.85 34.84,19.34 34.84,1.56 32.3,-0.98
  pour Bottom: 0.55,-1.23 -0.97,0.29 -0.97,19.09 -0.97,19.34 -0.72,19.59 34.08,19.59 34.59,19.09 34.59,1.56 31.79,-1.23
ILM
  Top 0.152: U6.12 24.53,5.51 24.53,4.07 R3.2
ISET
  Top 0.152: U6.16 26.4,4.66 26.92,4.14 R4.2
LED1
  Top 0.152: R5.2 28.4,22.56 LED1.A
LED2
  Top 0.152: R8.2 26.08,23.55 LED2.A
LED3
  Top 0.152: R9.2 26.08,24.51 LED3.A
NFC1  (via drill 0.2)
  Top 0.152: U2.7 10.67,11.24 11.02,11.59 11.02,14.78 v10.99,14.8
  Bottom 0.152: v10.99,14.8 | v10.99,14.8 10.99,15.03 11.95,15.99 11.95,17.56 10.49,19.03 NFC2.TP
NFC2  (via drill 0.2)
  Top 0.152: U2.8 10.63,10.14 10.81,10.33 10.81,10.95 11.65,11.78 v11.65,14.87
  Bottom 0.152: v11.65,14.87 11.7,14.87 12.28,15.45 12.28,19.23 NFC1.TP
P2_AIN0
  Top 0.152: U2.5 9.44,13.16 8.68,13.16 8.63,13.11 X3.16
P3_AIN1
  Top 0.152: U2.6 9.45,12.07 8.87,12.07 8.65,11.85 8.64,11.84 X3.18
P4_AIN2
  Top 0.152: U2.A3 13.72,13.44 13.19,13.97 12.89,13.97 12.44,14.43 12.44,15.19 12.14,15.5 12.14,17.31 10.59,18.85 10.05,18.85 8.17,20.73 X3.4
P5_AIN3
  Top 0.152: U2.A4 13.72,12.24 13.19,12.77 12.75,12.77 12.44,12.46 12.44,12.15 11.22,10.93 11.22,9.9 10.84,9.52 8.7,9.52 7.64,10.57 X3.20
P7
  Top 0.152: U2.A5 13.85,11.04 13.25,10.45 12.82,10.45 12.44,10.06 12.44,9.39 11.34,8.29 8.2,8.29 7.49,9 5.62,9 4.85,9.77 4.85,11.9 4.54,12.22 4.54,13.03 4.23,13.33 4.23,14.27 3.93,14.57 3.93,15.31 3.62,15.62 3.62,16.4 3.32,16.71 3.32,17.62 3.01,17.92 3.01,18.74 2.29,19.46 X3.5
P11
  Top 0.152: U2.11 23.9,12.53 25.9,12.53 X4.15
P12
  Top 0.152: U2.E6 19.94,10.37 19.94,12.46 20.25,12.77 20.85,12.77 21.89,13.81 21.89,14.49 21.72,14.66 21.72,15.46 22.61,16.35 22.61,18.39 22.7,18.48 23.9,18.48 | 23.9,18.48 | 23.9,18.48 23.9,18.49 24.26,18.49 24.49,18.72 24.49,19.37 25.3,20.18 X4.3
P13
  Top 0.152: U2.13 23.99,14.81 25.64,14.81 X4.11
P16  (via drill 0.2)
  Top 0.152: U2.D3 18.97,13.24 v18.42,12.7 | v18.49,3.06 20.34,3.06 20.91,2.5 21.33,2.5 22.03,1.8 22.03,1.37 22.42,0.98 | 22.42,0.98 22.48,0.93 | 22.42,0.98 22.55,0.98 23.12,0.41 28.41,0.41 v29.09,1.09 | v30.19,17.53 30.31,17.64 X4.8
  Bottom 0.152: v18.42,12.7 18.42,11.96 18.1,11.64 18.1,11.33 16.8,10.03 15.58,10.03 15.48,10.13 15.08,10.13 14.01,9.06 14.01,7.23 14.75,6.5 15.15,6.5 15.76,7.11 16.74,7.11 18.07,5.78 18.07,3.66 18.49,3.24 v18.49,3.06 | v29.09,1.09 29.09,1.16 30.86,2.92 30.86,16.87 v30.19,17.53
P17  (via drill 0.2)
  Top 0.152: U2.C3 17.47,13.89 16.93,14.43 16.93,15.18 16.5,15.62 16.5,16.06 16.17,16.39 15.61,16.39 15.36,16.64 15.36,17.35 15.62,17.6 v15.62,17.69 | v30.22,16.56 30.4,16.37 X4.10
  Bottom 0.152: v15.62,17.69 15.62,17.97 15.98,18.34 28.47,18.34 30.25,16.56 v30.22,16.56
P20  (1 unrouted)
  Top 0.152: U2.E1 20.47,15.9 21.7,17.13 21.7,18.89 22.21,19.4 23.55,19.4 23.58,19.43 23.58,19.76 23.88,20.06 23.88,20.97 24.19,21.27 24.19,23.99 24.7,24.5
P21  (1 unrouted)
  Top 0.152: U2.E2 20.47,15.08 22,16.61 22,18.75 22.34,19.1 23.71,19.1 23.88,19.27 23.88,19.63 24.19,19.93 24.19,20.83 24.49,21.14 24.49,23.31 24.75,23.57
P22  (via drill 0.2)
  Top 0.152: U2.C2 17.47,15.07 16.8,15.74 16.8,16.19 16.5,16.49 16.5,17.71 v16.61,17.81 | v30.2,15.19 30.29,15.1 X4.12
  Bottom 0.152: v16.61,17.81 16.83,18.03 27.36,18.03 v30.2,15.19
P24  (via drill 0.2)
  Top 0.152: v17.89,16.43 17.89,16.26 U2.C1 | v30.16,12.84 30.43,12.56 X4.16
  Bottom 0.152: v17.89,16.43 17.89,17.2 18.1,17.41 25.58,17.41 v30.16,12.84
P25  (via drill 0.2)
  Top 0.152: v14.96,17.63 15.04,17.54 15.04,16.44 15.64,15.84 U2.B1 | v14.96,17.63 | v27.75,19.05 27.75,21.93 27.58,22.1 26.02,22.1 25.69,22.42 R5.1
  Bottom 0.152: v14.96,17.63 14.96,18.24 15.36,18.64 27.34,18.64 v27.75,19.05
P26_SDA
  Top 0.152: U2.1 9.67,17.9 8.6,17.9 8.3,18.19 X3.8
P27_SCL
  Top 0.152: U2.2 9.63,16.83 8.61,16.83 8.53,16.92 X3.10
P28_AIN4  (via drill 0.2)
  Top 0.152: U2.A1 13.94,16.38 v13.94,17.56 | v30.22,19.12 31.63,19.12 X4.6
  Bottom 0.152: v13.94,17.56 13.94,19.07 14.11,19.25 26.42,19.25 27.27,20.1 29.25,20.1 v30.23,19.12 v30.22,19.12
P30_AIN6  (via drill 0.2)
  Top 0.152: v30.15,14.01 30.32,13.83 X4.14 | U2.B2 15.38,15.23 14.2,15.23 v13.72,15.71
  Bottom 0.152: v30.15,14.01 26.44,17.72 17.2,17.72 16.43,16.95 14.83,16.95 13.72,15.85 v13.72,15.71
P31_AIN7
  Top 0.152: U2.B3 15.97,12.99 15.44,12.46 15.44,11.93 15.08,11.57 12.75,11.57 12.6,11.42 12.58,11.42 11.83,10.67 11.83,9.65 11.09,8.9 8.45,8.9 7.74,9.61 5.87,9.61 5.46,10.02 5.46,12.17 5.17,12.47 5.17,13.27 4.84,13.59 4.84,14.55 4.54,14.85 4.54,15.61 4.23,15.91 4.23,16.7 3.93,17 3.93,17.94 3.62,18.25 3.62,19.11 3.32,19.41 3.32,20.18 3.01,20.49 3.01,21.4 2.41,22 X3.1
P100
  Top 0.152: U2.12 24.14,13.44 24.38,13.68 25.79,13.68 X4.13
P103
  Top 0.152: U2.B6 15.96,9.34 15.74,9.11 14.88,9.11 14.68,9.31 13.71,9.31 11.78,7.37 7.82,7.37 7.11,8.09 5.24,8.09 3.94,9.39 3.94,11.47 3.62,11.79 3.62,12.63 3.32,12.94 3.32,13.87 3.01,14.17 3.01,14.86 2.22,15.65 X3.11
P104
  Top 0.152: U2.C6 17.47,9.51 15.52,7.56 12.87,7.56 12.07,6.75 7.58,6.75 6.86,7.48 4.99,7.48 3.32,9.14 3.32,11.21 3.01,11.52 3.01,12.37 2.27,13.11 X3.15
P105  (via drill 0.2)
  Top 0.152: 18.91,9.84 U2.D6 18.68,9.84 16.99,8.15 16.99,6.27 16.55,5.83 13.16,5.83 v12.66,5.32 | v10.32,3.86 v10.32,3.85 6.77,3.85 JP1.1
  Bottom 0.152: v12.66,5.32 11.19,3.86 v10.32,3.86
P106
  Top 0.152: U2.Z6 12.97,9.49 11.47,7.99 8.07,7.99 7.36,8.7 5.49,8.7 4.55,9.64 4.55,11.77 4.23,12.08 4.23,12.9 3.93,13.2 3.93,14.13 3.62,14.44 3.62,15.17 3.32,15.47 3.32,16.27 3.01,16.57 3.01,17.44 2.26,18.19 X3.7
P107  (via drill 0.2)
  Top 0.152: U2.E0 20.47,17 19.83,17 v19.74,16.91 | v30.17,11.78 30.65,11.29 X4.18
  Bottom 0.152: v30.17,11.78 24.85,17.09 19.92,17.09 v19.74,16.91
P108
  Top 0.152: U2.A6 13.78,9.84 11.62,7.68 7.95,7.68 7.24,8.39 5.36,8.39 4.24,9.51 4.24,11.64 3.93,11.96 3.93,12.77 3.62,13.07 3.62,14.01 3.32,14.31 3.32,15 3.01,15.31 3.01,16.13 2.83,16.31 2.22,16.92 X3.9
P109
  Top 0.152: U2.E3 20.56,13.53 21.07,13.53 21.57,14.03 21.57,14.36 21.4,14.52 21.4,15.58 22.31,16.48 22.31,18.63 22.47,18.79 24.14,18.79 24.19,18.84 24.19,19.5 24.49,19.81 24.49,20.65 25.3,21.46 X4.1
P110  (1 unrouted)
  Top 0.152: 12.87,11.04 U2.Z5 12.97,11.02 12.14,10.19 12.14,9.52 11.22,8.6 8.65,8.6 8.32,8.6 7.61,9.31 5.74,9.31 5.16,9.89 5.16,12.04 4.86,12.33 4.86,13.14 4.54,13.46 4.54,14.41 4.23,14.72 4.23,15.46 3.93,15.76 3.93,16.53 3.62,16.84 3.62,17.75 3.32,18.06 3.32,18.92 3.01,19.23 3.01,20.01 2.29,20.73 X3.3
P111  (via drill 0.2)
  Top 0.152: U2.Z0 12.97,17.6 v12.83,17.74 | v30.22,21.23 30.44,21.45 X4.2
  Bottom 0.152: v12.83,17.74 12.83,18.17 13.15,18.49 13.15,19.4 13.61,19.86 26.14,19.86 27.51,21.23 v30.22,21.23 30.23,21.23
P112  (via drill 0.2)
  Top 0.152: U2.Z1 12.97,16.03 v13.37,16.44 v13.37,16.45 | v30.14,20.36 31.66,20.36 X4.4
  Bottom 0.152: v13.37,16.45 13.46,16.53 13.46,19.26 13.76,19.56 26.26,19.56 27.3,20.59 29.91,20.59 v30.14,20.36
P113
  Top 0.152: U2.Z2 12.97,15.09 12.44,15.62 12.44,17.44 10.72,19.16 10.27,19.16 9.06,20.37 9.06,21.23 8.28,22 X3.2
P114
  Top 0.152: U2.Z3 12.13,14.28 12.13,15.07 11.81,15.39 11.81,17.18 10.46,18.53 9.19,18.53 8.25,19.46 X3.6
P115
  Top 0.152: U2.Z4 11.53,10.8 11.53,9.77 10.97,9.21 8.57,9.21 7.87,9.92 6,9.92 5.77,10.15 5.77,12.31 5.47,12.61 5.47,13.48 5.19,13.75 5.19,14.74 6.1,15.65 X3.12
PGOOD  (via drill 0.2)
  Top 0.152: U6.7 25.4,8.46 26.02,9.08 v26.02,9.19 | v19.75,15.92 19.94,15.73 19.94,15.33 19.25,14.64 U2.D2 | v27.6,10.76 27.6,12.54 v27.62,12.56
  Bottom 0.152: v26.02,9.19 26.02,9.44 R10.2 26.18,10.22 26.56,10.61 27.32,10.61 27.47,10.76 v27.6,10.76 | v19.75,15.92 19.78,15.96 24.28,15.96 27.62,12.62 v27.62,12.56
RESET  (via drill 0.2)
  Top 0.152: v22.53,13.31 22.74,13.52 22.74,15 23.39,15.64 U2.14 24.36,15.64 25.1,16.37 X4.9
  Bottom 0.152: R2.1 23.65,13.58 22.8,13.58 v22.53,13.31
SCLK  (via drill 0.2)  (1 unrouted)
  Top 0.152: X3.13 2.36,14.38 3.01,13.74 3.01,12.81 3.32,12.5 3.32,11.65 3.63,11.34 3.63,9.27 5.11,7.78 6.98,7.78 7.7,7.06 11.92,7.06 13.64,8.78 v14.49,8.78 14.49,8.81 15.88,8.81 16.63,9.56 16.63,10.22 16.94,10.53 16.94,11.39 17.47,11.92 U2.C4
  Bottom 0.152: v14.49,8.78 14.88,9.16 18.03,9.16
SWDCLK
  Top 0.152: U2.15 24.17,16.74 25.07,17.64 X4.7
SWDIO
  Top 0.152: U2.16 24.05,17.84 25.12,18.91 X4.5
SYNC/RESET  (via drill 0.2)
  Top 0.152: U2.B5 16.03,11.04 16.03,10.71 v16.23,10.51
  Bottom 0.152: U5.16 17.02,11.61 17.02,10.68 16.77,10.43 16.31,10.43 v16.23,10.51 | v16.23,10.51
TS
  Top 0.152: R1.2 27.54,4.8 27.54,5.75 27.47,5.82 U6.1
VDD  (via drill 0.2)
  Top 0.152: 23.68,8.86 C12.2 | U2.9 23.68,10.1 23.68,8.86 | U2.F4 21.97,12.06 22.72,11.31 22.72,10.67 23.25,10.14 U2.9 | 23.68,9.21 v23.68,9.3 23.68,8.86 | v24.67,9.21 23.73,10.14 U2.9 | v22.73,7.09 22.73,7.67 U3.5 22.4,8.02 23.06,8.67 C12.2 | U2.9 23.82,10.04 25,10.04 25.02,10.02 X4.19 | 23.68,8.86 C12.2
  Bottom 0.152: U5.26 16.53,6.18 17.24,6.18 17.39,6.03 17.39,5.94 17.39,4.03 C23.2 17.37,3.56 17.37,2.47 17.93,1.92 22.45,1.92 23.56,3.03 23.56,6.34 23.32,6.58 23.17,6.58 22.73,7.01 v22.73,7.09 | v22.73,7.09 22.73,6.98 | R13.2 21.11,12.19 22.35,10.96 22.45,10.96 C15.2 23.5,10.82 23.68,10.64 v23.68,9.3 | R2.2 23.71,12.96 24.43,12.24 C22.2 | C22.2 24.5,11.25 24.5,9.38 v24.67,9.21 | R11.1 24.08,7.08 23.61,7.55 23.18,7.55 v22.73,7.1 v22.73,7.09 | R10.1 24.41,11.32 C22.2
VIN  (via drill 0.2)
  Top 0.152: S1.2 18.48,5.24 | S1.2 18.17,7.48 C13.2 19.85,7.94 U3.1 | 20.36,6.09 U3.3 19.88,6.07 19.88,4.38 19.65,4.15 18.35,4.15 18.17,4.32 S1.2 | 20.23,7.99 U3.1 | v19.86,13.08 19.86,12.89 19.63,12.66 19.63,8.25 U3.1 | v18.23,15.82 18.14,15.74 v18.14,14.33
  Bottom 0.152: v19.86,13.08 19.49,13.08 U4.3 | U4.1 19.32,15.16 18.9,15.16 v18.23,15.82 | U4.3 18.84,13.73 18.56,13.73 18.37,13.92 18.37,14.09 v18.14,14.33 | C7.1 19.45,13.49 U4.3
VSWITCH  (via drill 0.2)
  Top 0.152: 23.86,6.54 23.86,6.82 U6.10 | 23.86,6.54 23.86,6.32 U6.11 | v24.04,4.66 24.04,5.12 23.55,5.61 23.55,6.44 | S1.3 19.72,1.04 v19.66,1.1 | U6.5 26.47,8.01 26.88,8.42 v27.58,8.42 | v23.4,7.06 23.4,6.94 23.55,6.78 23.55,6.44 | 23.86,6.54 23.75,6.44 23.55,6.44
  Bottom 0.152: v24.04,4.66 24.04,3.02 22.61,1.59 20.15,1.59 v19.66,1.1 | v23.4,7.06 23.4,6.95 24.92,5.42 26.52,5.42 27.29,6.18 27.29,8.12 v27.58,8.42 27.49,8.52 C11.2
XTAL1_1  (via drill 0.2)
  Top 0.152: v10.94,17.23 10.94,16.53 10.05,15.64 U2.3
  Bottom 0.152: v10.94,17.23 10.39,16.68 X2.2 7.28,16.59 C2.2
XTAL2_1  (via drill 0.2)
  Top 0.152: v10.93,15.84 10.7,15.6 10.7,15.19 10.05,14.54 U2.4
  Bottom 0.152: v10.93,15.84 10.33,15.23 7.62,15.23 X2.1 7.35,14.96 C1.2

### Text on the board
tPlace: BT840, BT40, / or Other BT-Series Footprints | I1
bPlace: BT(8)40 + ADS131M08 / JOSHUA BREWSTER / BOJAN JOVANOVICH / AGPL v3 LICENSE
tNames: P105
bNames: SWDIO | SWDCLK | RESET | 7+ | 7- | GND | 3.3V | 0+ | 0-
tValues: G | V
Document: RESET | SWDIO | SWO | SWDCLK | GND | VDD

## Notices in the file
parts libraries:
spkfncoils: Licensing: Creative Commons ShareAlike 4.0 International - https://creativecommons.org/licenses/by-sa/4.0
